(* Logix 5000 AddOnInstructionDefinition export; software revision 16.00 *)

ADD_ON_INSTRUCTION SCLR   (* revision 1.0, vendor Rockwell Automation *)
// Scale with Rate
// Help:
// All information provided "AS IS" - No Warranty or implied merchantability.
// Refer to the RSLogix 5000 End User License Agreement (EULA) in the Release Notes
// This routine performs the operation of the SLC-500 Scale With Parameters instruction (SCL).
// Description:
// Use this instruction to scale data from your analog module and bring it into the limits prescribed by the process variable or another analog module. For example, use SCL to convert a 4-20 mA input signal to a PID process variable. Or use SCL to scale an analog input to control an analog output.
// When rung conditions are true, this instruction multiplies the source by a specified rate. The rounded result is added to an offset value and placed in the destination.
// Equations used in calculating a linear relationship:
// Scaled value = (input value x rate) + offset
// Rate = (scaled max. - scaled min.) / (input max. - input min.)
// Offset = scaled minimum - (input minimum x rate)
VAR_INPUT
   Source : REAL; {required}   // Input Value to be scaled
   Rate : REAL; {required}   // +/- value multiplied against source to represent the rate of change or slop of the desired output range
   Offset : REAL; {required}   // +/- Value to adjust result after rate is applied
END_VAR
VAR_OUTPUT
   Destination : REAL; {required}   // Resulting Scaled Value
END_VAR
VAR
   Temp : REAL;
END_VAR

ROUTINE Logic   (* ladder *)
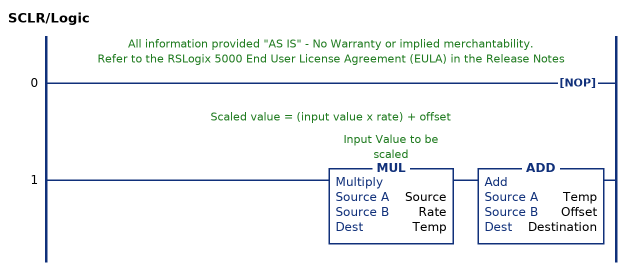
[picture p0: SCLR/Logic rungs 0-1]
   // All information provided "AS IS" - No Warranty or implied merchantability.
   // Refer to the RSLogix 5000 End User License Agreement (EULA) in the Release Notes
   0: NOP();
   // Scaled value = (input value x rate) + offset
   1: MUL(Source,Rate,Temp)ADD(Temp,Offset,Destination);
END_ROUTINE
END_ADD_ON_INSTRUCTION
